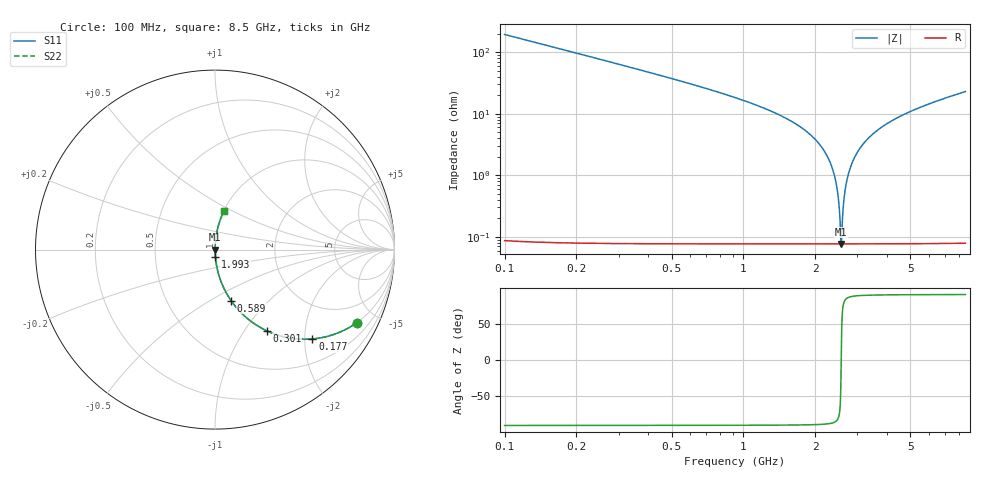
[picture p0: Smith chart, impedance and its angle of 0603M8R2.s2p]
! Created Wed Apr 18 16:33:50 2012
# hz S ma R 50
! 2 Port Network Data from SP1.SP block
! freq  magS11  angS11  magS21  angS21  magS12  angS12  magS22  angS22
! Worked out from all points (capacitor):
!   8401 points, 100 MHz to 8.5 GHz, reference 50 ohm
!   read as one part in series: C = 8.21 pF near 142 MHz
!   lowest |Z| = 76.9 mohm at 2.567 GHz (marker M1)
!   series resonance near 2.567 GHz, so ESL is about 470 pH
!   S11 on the Smith chart (normalised r, x): 100 MHz: 1.00, -3.87; 177 MHz: 1.00, -2.18; 301 MHz: 1.00, -1.27; 589 MHz: 1.00, -0.62; 1.993 GHz: 1.00, -0.08; 8.5 GHz: 1.00, +0.46
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1e8  0.8883 -27.3  0.4589 62.7  0.4589 62.7  0.8883 -27.3
1.77e8  0.7366 -42.5  0.6758 47.4  0.6758 47.4  0.7366 -42.5
3.01e8  0.5359 -57.5  0.8436 32.4  0.8436 32.4  0.5359 -57.5
5.89e8  0.2975 -72.6  0.954 17.3  0.954 17.3  0.2975 -72.6
1.5e9  0.08477 -84.6  0.9956 4.9  0.9956 4.9  0.08477 -84.6
1.993e9  0.03861 -86.6  0.9985 2.2  0.9985 2.2  0.03861 -86.6
2.226e9  0.02161 -86.7  0.999 1.2  0.999 1.2  0.02161 -86.7
2.384e9  0.01121 -85.4  0.9992 0.6  0.9992 0.6  0.01121 -85.4
2.472e9  0.005756 -82.0  0.9992 0.3  0.9992 0.3  0.005756 -82.0
2.541e9  0.001726 -63.5  0.9992 0.1  0.9992 0.1  0.001726 -63.5
2.567e9  0.0007681 -0.6  0.9992 0.0  0.9992 0.0  0.0007681 -0.6
2.591e9  0.001594 61.1  0.9992 -0.1  0.9992 -0.1  0.001594 61.1
2.642e9  0.004409 79.7  0.9992 -0.2  0.9992 -0.2  0.004409 79.7
2.697e9  0.007495 83.7  0.9992 -0.4  0.9992 -0.4  0.007495 83.7
2.782e9  0.01218 85.7  0.9992 -0.7  0.9992 -0.7  0.01218 85.7
2.9e9  0.01847 86.6  0.9991 -1.1  0.9991 -1.1  0.01847 86.6
3.115e9  0.0294 86.8  0.9988 -1.7  0.9988 -1.7  0.0294 86.8
3.41e9  0.04345 86.5  0.9983 -2.5  0.9983 -2.5  0.04345 86.5
4.3e9  0.08124 84.8  0.9959 -4.7  0.9959 -4.7  0.08124 84.8
5.7e9  0.1329 82.0  0.9904 -7.6  0.9904 -7.6  0.1329 82.0
7.1e9  0.1795 79.4  0.983 -10.3  0.983 -10.3  0.1795 79.4
8.5e9  0.2232 76.9  0.974 -12.9  0.974 -12.9  0.2232 76.9
